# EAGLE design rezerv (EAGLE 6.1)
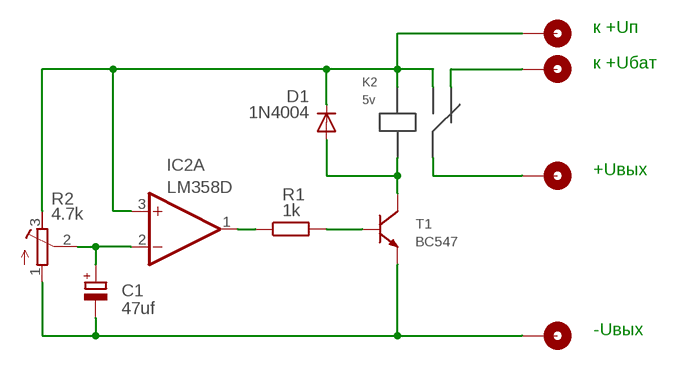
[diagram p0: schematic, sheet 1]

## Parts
C1  47uf  CPOL-EUE2.5-7  [E2,5-7]
D1  1N4004  [DO41-10]
IC2  LM358D  [SO08]
K2  5v  HK4100FHK4100F  [HK4100F]
PIN1  PINPIN  [PIN]
PIN2  PINPIN  [PIN]
PIN3  PINPIN  [PIN]
PIN5  PINPIN  [PIN]
R1  1k  R-EU_0207/10  [0207/10]
R2  4.7k  R-TRIMM64Y  [RTRIM64Y]
T1  BC547  [BC547]

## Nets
N$1: D1.A K2.R2(K2) T1.K
N$2: R1.2 T1.B
N$3: IC2.1(A:OUT) R1.1
N$4: K2.P1 PIN2.P$1
N$5: D1.C IC2.3(A:+IN) K2.K1 K2.NO PIN5.P$1 R2.3(E)
N$6: C1.- PIN1.P$1 R2.1(A) T1.E
N$7: C1.+ IC2.2(A:-IN) R2.2(S)
N$8: K2.NC PIN3.P$1
Unconnected: IC2.5(B:+IN) IC2.6(B:-IN) IC2.7(B:OUT)

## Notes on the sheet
- к +Uп
- к +Uбат
- +Uвых
- -Uвых

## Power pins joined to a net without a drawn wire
V+: IC2.8(P:V+)
V-: IC2.4(P:V-)

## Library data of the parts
C1 = rcl:CPOL-EU: POLARIZED CAPACITOR, European symbol
D1 = diode:1N4004: DIODE
IC2 = linear:LM358: OP AMP also LM158; LM258; LM2904 Source: http://cache.national.com/ds/LM/LM158.pdf
K2 = untitled:HK4100F
PIN1-PIN3 PIN5 = untitled:PIN
R1 = rcl:R-EU_: RESISTOR, European symbol
R2 = rcl:R-TRIMM: Trimm resistor
T1 = untitled:BC547

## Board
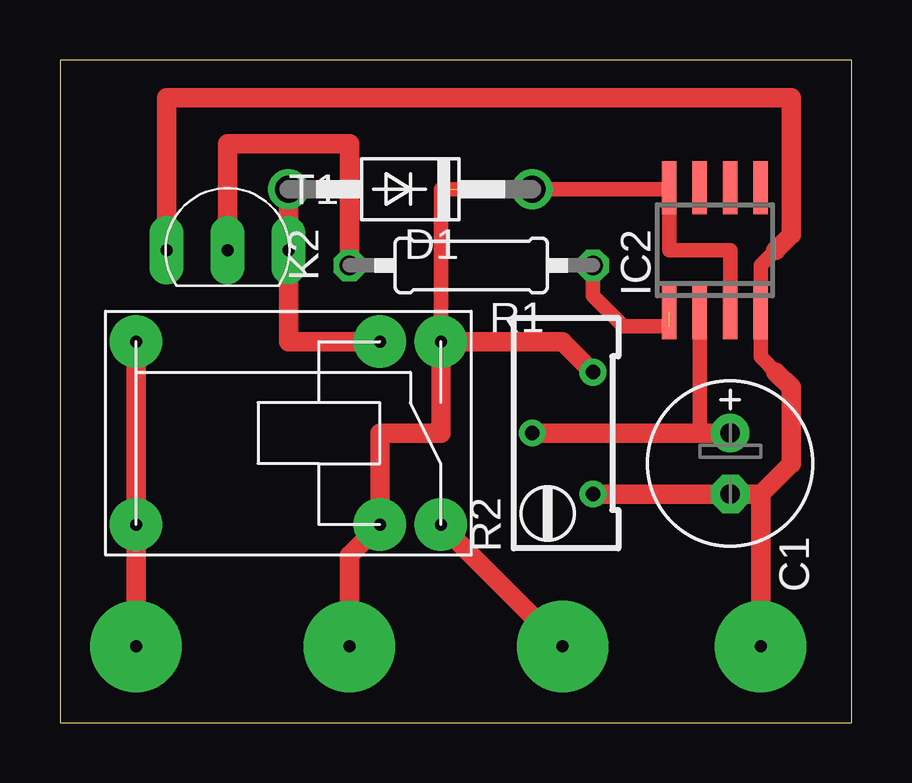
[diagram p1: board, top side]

Size 33 x 27.61 mm. Coordinates in mm from the lower left corner, seen from the top.
Outline: 0,0 33,0 33,27.61 0,27.61 0,0
Copper layers (1*16): Top 0.035mm / dielectric 1.5mm / Bottom 0.035mm
Design rules: minimum track width 10mil, minimum drill 24mil, track to track 8mil, track to pad 8mil, pad to pad 8mil, via to via 8mil, smd to smd 8mil, copper to edge 40mil, drill to drill 8mil, minimum pad ring 10mil, minimum via ring 8mil, stop-mask expansion 4mil, vias tented up to drill 0mil, thermal gap 10mil

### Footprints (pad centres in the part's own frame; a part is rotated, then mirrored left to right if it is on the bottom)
E2,5-7 = drill 0.813 pad 1.6: + -1.27,0 | drill 0.813 pad 1.6 octagon: - 1.27,0
DO41-10 = drill 1.118: A 5.08,0; C -5.08,0
SO08 = smd 0.6 x 2.2: 1 -1.905,-2.6; 2 -0.635,-2.6; 3 0.635,-2.6; 4 1.905,-2.6; 5 1.905,2.6; 6 0.635,2.6; 7 -0.635,2.6; 8 -1.905,2.6
HK4100F = drill 0.5 pad 2.184: K1 -3.81,-8.89; NC 3.81,1.27; NO 3.81,-11.43; P1 -3.81,-11.43; P$1 -3.81,1.27; R2 3.81,-8.89
PIN = drill 0.5 pad 3.81: P$1 0,0
0207/10 = drill 0.813 octagon: 1 -5.08,0; 2 5.08,0
RTRIM64Y = drill 0.61: 1 0,-2.54; 2 -2.54,0; 3 0,2.54
BC547 = drill 0.5 pad 1.422 long: B 0,0; E -2.54,0; K 2.54,0

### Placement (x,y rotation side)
C1  27.94,10.79 270 top
D1  14.61,22.23 180 top
IC2  27.3,19.68 0 top
K2  4.45,12.06 90 top
PIN1  29.21,3.17 0 top
PIN2  20.95,3.17 0 top
PIN3  3.17,3.17 0 top
PIN5  12.06,3.17 0 top
R1  17.14,19.05 180 top
R2  22.23,12.06 0 top
T1  6.99,19.68 0 top

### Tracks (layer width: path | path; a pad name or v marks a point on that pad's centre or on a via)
N$1
  Top 0.813: K2.R2 9.53,15.88 T1.K D1.A
N$2
  Top 0.813: T1.B 6.99,24.13 12.06,24.13 R1.2
N$3  (1 unrouted)
  Top 0.61: R1.1 22.23,17.78 23.5,16.51 25.4,16.51
N$4
  Top 0.813: K2.P1 PIN2.P$1
N$5  (1 unrouted)
  Top 0.61: IC2.3 27.94,19.68 25.4,19.68 25.4,22.23 15.88,22.23 K2.NO
  Top 0.813: PIN5.P$1 12.06,6.99 K2.K1 13.34,12.06 15.88,12.06 K2.NO 20.95,15.88 R2.3
N$6
  Top 0.61: 29.84,14.61 29.21,15.24 29.21,19.05 29.84,19.68
  Top 0.813: 29.21,9.53 PIN1.P$1 | R2.1 C1.- 29.21,9.53 | 29.21,9.53 30.48,10.79 30.48,13.97 29.84,14.61 | T1.E 4.45,26.04 30.48,26.04 30.48,20.32 29.84,19.68
N$7
  Top 0.61: IC2.2 26.67,12.06 C1.+
  Top 0.813: R2.2 C1.+
N$8
  Top 0.813: PIN3.P$1 K2.NC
